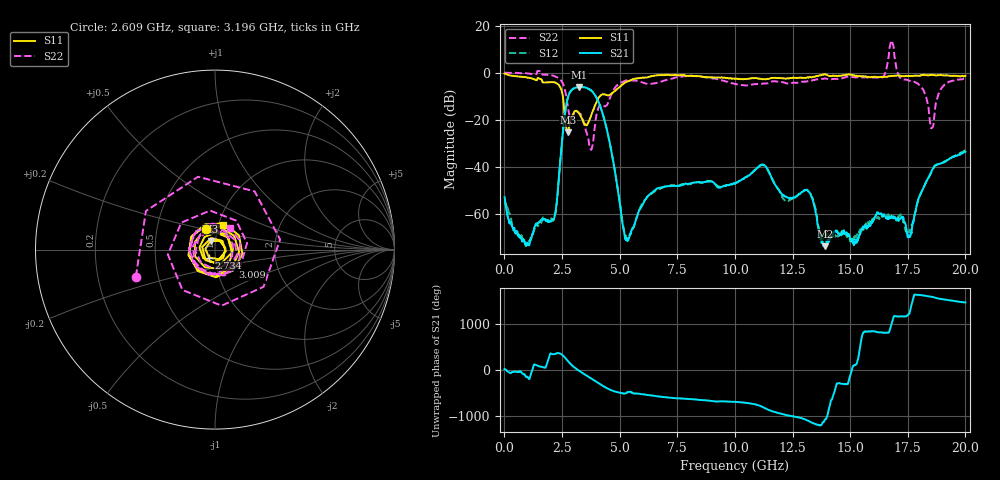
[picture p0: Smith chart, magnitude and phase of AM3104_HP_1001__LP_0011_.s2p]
!Created with skrf (http://scikit-rf.org).
# Hz S RI R 50.0
!freq ReS11 ImS11 ReS21 ImS21 ReS12 ImS12 ReS22 ImS22
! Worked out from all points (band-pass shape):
!   1601 points, 10 MHz to 20 GHz, reference 50 ohm
!   highest |S21| = -6.08 dB at 3.258 GHz (marker M1); lowest = -73.8 dB at 13.93 GHz (marker M2)
!   |S21| within 3 dB of the highest: 2.806 GHz to 3.901 GHz (1.095 GHz wide, 32.7 % of centre)
!   lowest |S11| = -25.4 dB at 2.759 GHz (marker M3), VSWR 1.11, Z = 47.4 + j4.51 ohm
!   |S11| at or under -10 dB: 2.536 GHz to 4.15 GHz (1.615 GHz wide, 48.3 % of centre)
!   |S22| runs from -32.8 to 13.7 dB; largest |S21 - S12| = 0.025
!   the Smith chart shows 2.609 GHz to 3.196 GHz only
!   S11 on the Smith chart (normalised r, x): 2.609 GHz: 0.88, +0.21; 2.734 GHz: 0.93, -0.08; 3.009 GHz: 1.19, -0.24; 3.196 GHz: 1.05, +0.29
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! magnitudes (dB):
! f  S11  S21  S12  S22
! 10 MHz  -0.4  -53.0  -54.7  -0.1
! 997 MHz  -2.1  -73.5  -72.6  -0.4
! 2.084 GHz  -4.0  -62.8  -62.4  -1.2
! 2.609 GHz  -18.1  -19.1  -19.1  -6.6
! 2.734 GHz  -25.1  -11.4  -11.4  -13.2
! 2.759 GHz  -25.4  -10.5  -10.5  -14.8
! 3.009 GHz  -17.2  -6.7  -6.7  -17.7
! 3.196 GHz  -16.8  -6.2  -6.2  -16.8
! 3.258 GHz  -17.6  -6.1  -6.2  -17.5
! 3.346 GHz  -19.1  -6.1  -6.2  -18.3
! 3.758 GHz  -18.4  -7.5  -7.6  -32.8
! 4.27 GHz  -9.2  -17.7  -17.7  -13.7
! 5.295 GHz  -4.0  -71.2  -70.5  -3.3
! 6.682 GHz  -1.1  -49.1  -49.5  -4.2
! 10.01 GHz  -2.7  -47.2  -47.2  -4.8
! 11.2 GHz  -2.8  -39.1  -39.3  -4.7
! 13.34 GHz  -2.0  -53.2  -53.0  -3.4
! 13.93 GHz  -0.7  -73.8  -68.8  -2.5
! 16.68 GHz  -1.5  -62.0  -60.9  7.2
! 17.58 GHz  -1.4  -69.8  -67.4  -3.5
! 18.54 GHz  -0.9  -41.8  -42.0  -23.6
! 20 GHz  -1.4  -33.7  -33.0  -2.5
